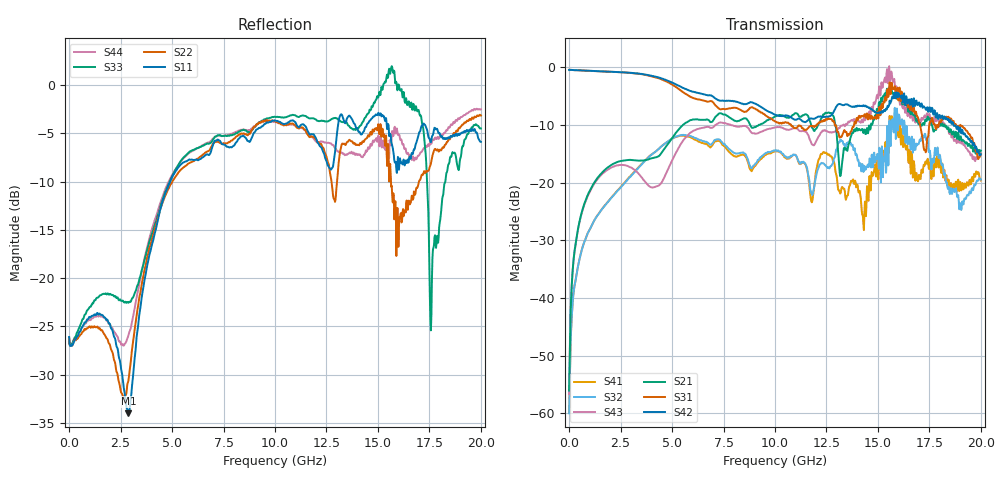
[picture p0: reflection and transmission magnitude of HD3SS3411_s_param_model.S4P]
!  4-Port S-parameters saved by WinCal
! VAR MeasName=S-Parameters (CALIBRATED_DATA) read from VNA (N5230A)
! VAR MeasDate=1/22/2015 10:09:58 AM
! VAR NAME=HD3SS3411_A_to_B_SEL_L
! VAR FILENAME=HD3SS3411_A_to_B_SEL_L.S4P
! VAR DATE=1/22/2015 10:09:58 AM
! VAR PHYS_PORTS=1,2,3,4
! VAR ObjTypeName=DATASET
! VAR IndexType=Frequency
# Hz S MA R 50
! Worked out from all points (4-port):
!   800 points, 300 kHz to 20 GHz, reference 50 ohm
!   strongest paths, dB at 300 kHz, 5.006 GHz, 10.01 GHz, 15.02 GHz, 20 GHz:
!     S42: -0.5, -2.7, -8.3, -7.9, -15.1
!     S31: -0.5, -3.0, -9.4, -8.9, -15.0
!     S21: -56.0, -12.3, -8.6, -7.6, -14.5
!     S43: -56.6, -16.1, -10.4, -5.3, -14.9
!     S32: -60.0, -12.4, -14.4, -16.1, -19.5
!     S41: -59.9, -12.4, -14.6, -19.5, -19.6
!   lowest |S11| = -34.0 dB at 2.879 GHz (marker M1), VSWR 1.04, Z = 49.5 - j1.93 ohm
!   |S11| at or under -10 dB: start of sweep to 4.9 GHz
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300000  0.04954 -3.9  0.001492 -5.4  0.9454 0.5  0.0012 -4.3
        0.001579 -4.8  0.04902 -2.2  0.0009487 -13.3  0.9455 0.4
        0.9481 -0.2  0.001003 -10.0  0.04663 6.8  0.001461 3.1
        0.001017 -5.6  0.9452 0.4  0.001474 1.2  0.04964 -3.1
6.511038e8  0.05623 16.2  0.05831 69.3  0.9357 -18.0  0.02744 -119.2
            0.05844 69.3  0.05275 10.7  0.02746 -119.5  0.9362 -17.7
            0.9355 -18.1  0.02745 -119.6  0.06135 16.1  0.05742 67.1
            0.02751 -119.2  0.9358 -17.7  0.05744 67.2  0.05581 11.9
2.878855e9  0.01994 -102.6  0.1565 26.4  0.8942 -78.6  0.1092 -173.4
            0.1569 26.6  0.02938 -134.7  0.1081 -174.4  0.8954 -76.7
            0.895 -78.6  0.1081 -175.0  0.07458 -80.0  0.1383 12.9
            0.1093 -173.2  0.8943 -76.9  0.1384 12.9  0.05041 -109.5
1.078862e10  0.6549 -9.4  0.3512 -94.8  0.3059 106.5  0.162 -67.7
             0.3729 -93.8  0.6318 -1.8  0.1784 -66.0  0.3772 108.3
             0.3126 107.0  0.1709 -67.9  0.6985 -14.4  0.2893 -90.8
             0.1677 -65.9  0.3666 107.8  0.2899 -90.7  0.6242 -6.1
1.534425e10  0.6531 -104.1  0.5949 157.9  0.5215 55.1  0.1909 -96.5
             0.5941 147.5  0.4857 -152.4  0.2174 -143.1  0.4209 27.1
             0.5434 45.7  0.199 -131.8  1.045 -120.5  0.8072 138.4
             0.2031 -118.6  0.4156 23.4  0.8138 132.8  0.4632 -143.8
1.707138e10  0.5886 -120.6  0.3403 58.2  0.3285 -63.7  0.1233 144.5
             0.3197 60.3  0.328 -165.0  0.2364 121.8  0.4925 -51.1
             0.2988 -58.1  0.2295 125.3  0.6985 123.4  0.3517 51.8
             0.1073 150.8  0.4549 -46.8  0.3326 49.8  0.4486 165.3
2e10  0.5086 154.8  0.2005 -27.1  0.1803 -106.9  0.09519 50.0
      0.189 -25.8  0.697 119.3  0.1068 71.0  0.1596 -152.1
      0.177 -106.8  0.1062 69.4  0.5967 133.0  0.1602 -48.8
      0.1042 54.2  0.1763 -149.6  0.1792 -45.9  0.7492 111.7
